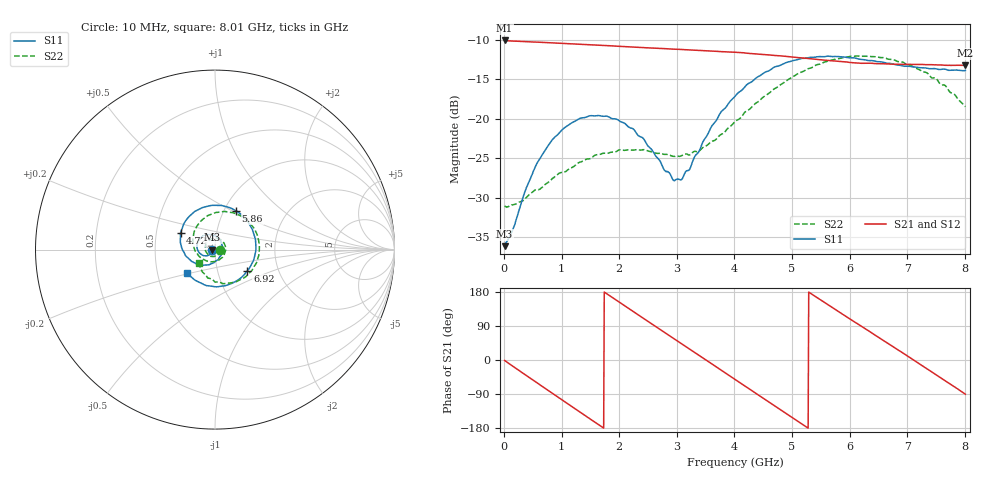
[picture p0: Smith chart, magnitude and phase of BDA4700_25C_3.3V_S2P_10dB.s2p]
!Agilent Technologies,E5071B,MY42404982,A.09.10
!Date: Mon Oct 20 18:07:12 2025
!Data & Calibration Information:
!Freq	S11:SOLT2(ON)	S21:SOLT2(ON)	S12:SOLT2(ON)	S22:SOLT2(ON)
# Hz S RI R 50
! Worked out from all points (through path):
!   801 points, 10 MHz to 8.01 GHz, reference 50 ohm
!   highest |S21| = -10.11 dB at 10 MHz (marker M1); lowest = -13.3 dB at 8.01 GHz (marker M2)
!   group delay of S21, straight-line fit = 280 ps
!   lowest |S11| = -36.1 dB at 10 MHz (marker M3), VSWR 1.03, Z = 48.5 - j0.123 ohm
!   |S11| at or under -10 dB: start of sweep to end of sweep
!   |S22| runs from -31.2 to -12.1 dB; largest |S21 - S12| = 0.0036
!   S11 on the Smith chart (normalised r, x): 10 MHz: 0.97, -0.00; 4.72 GHz: 0.67, +0.13; 5.86 GHz: 1.14, +0.52; 6.92 GHz: 1.39, -0.35; 8.01 GHz: 0.71, -0.19
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1e7  -0.0156 -0.00127  0.3121 -0.00679  0.312 -0.00725  0.0281 -0.0015
3.3e8  -0.0232 -0.022  0.252 -0.1762  0.2519 -0.1762  0.0222 -0.0207
7.2e8  -0.0534 -0.035  0.0755 -0.2934  0.0756 -0.2933  -0.00357 -0.0384
1.02e9  -0.0828 -0.0227  -0.0855 -0.2869  -0.0855 -0.2869  -0.0316 -0.0332
1.35e9  -0.1006 0.0115  -0.2283 -0.1873  -0.2284 -0.1875  -0.0535 -0.00292
1.64e9  -0.0927 0.0489  -0.2875 -0.0483  -0.2876 -0.0485  -0.0504 0.0314
1.93e9  -0.0637 0.0769  -0.27 0.0992  -0.2701 0.0992  -0.0231 0.0572
2.32e9  -0.00936 0.0784  -0.1418 0.2445  -0.1416 0.2445  0.0264 0.0579
2.68e9  0.0321 0.0456  0.031 0.2767  0.0307 0.2766  0.0571 0.0198
2.94e9  0.0406 0.0053  0.1488 0.2317  0.1486 0.2311  0.0558 -0.0155
3.08e9  0.0371 -0.018  0.2007 0.1863  0.1987 0.1876  0.0471 -0.0345
3.53e9  -0.0166 -0.0772  0.2684 -0.0113  0.2684 -0.0118  -0.0111 -0.0673
4.01e9  -0.1188 -0.0714  0.1647 -0.2049  0.1651 -0.2044  -0.0877 -0.038
4.37e9  -0.18 -0.00351  0.0104 -0.2567  0.0102 -0.2573  -0.1222 0.0275
4.72e9  -0.1917 0.0941  -0.1379 -0.2094  -0.137 -0.2101  -0.1119 0.1095
5.35e9  -0.0582 0.2374  -0.2372 0.0285  -0.2373 0.027  0.0291 0.2089
5.86e9  0.1166 0.2166  -0.1238 0.1936  -0.1236 0.1933  0.1834 0.1587
6.28e9  0.2113 0.1028  0.0308 0.2218  0.0338 0.2205  0.2464 0.0314
6.68e9  0.2196 -0.0421  0.1638 0.1492  0.1642 0.1489  0.2172 -0.0959
6.92e9  0.1802 -0.1186  0.2088 0.0716  0.2086 0.0703  0.1675 -0.1544
7.46e9  0.013 -0.2071  0.1797 -0.1255  0.1797 -0.1256  0.00701 -0.1808
8.01e9  -0.1537 -0.1308  -0.000777 -0.2172  -0.000281 -0.2173  -0.0919 -0.0758
